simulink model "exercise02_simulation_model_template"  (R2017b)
settings: Solver=ode45  StartTime=0.0  StopTime=10  FixedStep=1e-5  MaxStep=1e-3  RelTol=1e-4  EnableMultiTasking=on
InitFcn:
  | exercise02_simulation_parameters
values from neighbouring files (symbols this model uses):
  cmd_2_newtons_conversion_linear_coefficient = 6.4870e-6    (= 6.487e-06)    [exercise02_get_crazyflie_inner_controller.m]
  cmd_2_newtons_conversion_quadratic_coefficient = 1.3385e-10    [exercise02_get_crazyflie_inner_controller.m]
  cmd_max = 2^16-1    (= 65535)    [exercise02_get_crazyflie_inner_controller.m]
  cmd_min = 0    [exercise02_get_crazyflie_inner_controller.m]
  g = 9.81    [exercise02_get_crazyflie_vehicle_paramters.m]
  K_lqr_outer_loop = K_lqr_outer_loop_discrete_time_200Hz    [exercise02_simulation_parameters.m]
  measurement_noise_accelerometer_covariance_decomposition = U * sqrt(D)    [exercise02_get_measurement_noise_details.m]
  measurement_noise_accelerometer_mean = zeros(3,1)    [exercise02_get_measurement_noise_details.m]
  measurement_noise_accelerometer_seed = randi(measurement_noise_randStream_for_seeds,2^32-1,3,1)    [exercise02_get_measurement_noise_details.m]
  measurement_noise_accelerometer_var = measurement_noise_accelerometer_stddev.^2    [exercise02_get_measurement_noise_details.m]
  measurement_noise_body_accelerations_inclusion_multiplier = 0    [exercise02_get_measurement_noise_details.m]
  measurement_noise_body_rates_inclusion_multiplier = 0    [exercise02_get_measurement_noise_details.m]
  measurement_noise_full_state_covariance_decomposition = U * sqrt(D)    [exercise02_get_measurement_noise_details.m]
  measurement_noise_full_state_inclusion_multiplier = 0    [exercise02_get_measurement_noise_details.m]
  measurement_noise_full_state_mean = [         measurement_noise_p_mean        ;         measurement_noise_p_dot_mean    ;         measurement_noise_psi_mean      ;         measurement_noise_psi_dot_mean        ]    [exercise02_get_measurement_noise_details.m]
  measurement_noise_full_state_seed = [         measurement_noise_p_seed        ;         measurement_noise_p_dot_seed    ;         measurement_noise_psi_seed      ;         measurement_noise_psi_dot_seed        ]    [exercise02_get_measurement_noise_details.m]
  measurement_noise_gyroscope_covariance_decomposition = U * sqrt(D)    [exercise02_get_measurement_noise_details.m]
  measurement_noise_gyroscope_mean = zeros(3,1)    [exercise02_get_measurement_noise_details.m]
  measurement_noise_gyroscope_seed = randi(measurement_noise_randStream_for_seeds,2^32-1,3,1)    [exercise02_get_measurement_noise_details.m]
  measurement_noise_gyroscope_var = measurement_noise_gyroscope_stddev.^2    [exercise02_get_measurement_noise_details.m]
  nrotor_initial_condition = [         nrotor_initial_condition_p          ;         nrotor_initial_condition_p_dot      ;         nrotor_initial_condition_psi        ;         nrotor_initial_condition_psi_dot    ;     ]    [exercise02_get_crazyflie_vehicle_paramters.m]
  nrotor_vehicle_equilibrium_thrust = exercise02_compute_equilibrium_thrusts(nrotor_vehicle_layout_for_controller,nrotor_vehicle_mass_for_controller,g)    [exercise02_simulation_parameters.m]
  nrotor_vehicle_inertia_true = [         16.57 ,   0.83 ,   0.72 ;          0.83 ,  16.66 ,   1.80 ;          0.72 ,   1.80 ,  29.26       ] * 1e-6    [exercise02_get_crazyflie_vehicle_paramters.m]
  nrotor_vehicle_inertia_true_inverse = inv(nrotor_vehicle_inertia_true)    [exercise02_get_crazyflie_vehicle_paramters.m]
  nrotor_vehicle_layout_true = [         [  1 , -1 , -1 ,  1 ] * x_baseline  ;         [ -1 , -1 ,  1 ,  1 ] * y_baseline  ;         [ -1 ,  1 , -1 ,  1 ] * c_baseline        ]    [exercise02_get_crazyflie_vehicle_paramters.m]
  nrotor_vehicle_mass_true = 32e-3    (= 0.032)    [exercise02_get_crazyflie_vehicle_paramters.m]
  nrotor_vehicle_thrust_max = 0.1597*ones( size(nrotor_vehicle_layout_true,2) , 1 )    [exercise02_get_crazyflie_vehicle_paramters.m]
  pid_x_body_rate_integrator_limit = 33.3    [exercise02_get_crazyflie_inner_controller.m]
  pid_x_body_rate_kp = 250.0    (= 250)    [exercise02_get_crazyflie_inner_controller.m]
  pid_y_body_rate_integrator_limit = 33.3    [exercise02_get_crazyflie_inner_controller.m]
  pid_y_body_rate_kp = 250.0    (= 250)    [exercise02_get_crazyflie_inner_controller.m]
  pid_z_body_rate_kp = 120.0    (= 120)    [exercise02_get_crazyflie_inner_controller.m]
  reference_saw_tooth_amplitude_xyz_yaw = [0.3; 0.3; 0.3; 3*deg2rad]    [exercise02_get_reference_specification.m]
  reference_saw_tooth_bias_xyz_yaw = [0.0; 0.0; 0.0; 0*deg2rad]    [exercise02_get_reference_specification.m]
  reference_saw_tooth_inclusion_multiplier = 0    [exercise02_get_reference_specification.m]
  reference_sine_amplitude_xyz_yaw = [0.3; 0.3; 0.3; 3*deg2rad]    [exercise02_get_reference_specification.m]
  reference_sine_bias_xyz_yaw = [0.0; 0.0; 0.0; 0*deg2rad]    [exercise02_get_reference_specification.m]
  reference_sine_period = 5    [exercise02_get_reference_specification.m]
  reference_sine_wave_inclusion_multiplier = 0    [exercise02_get_reference_specification.m]
  reference_step_inclusion_multiplier = 0    [exercise02_get_reference_specification.m]
  reference_step_period = 5    [exercise02_get_reference_specification.m]
  reference_step_xyz_yaw = [0.5; 0.5; 0.5; 10*deg2rad]    [exercise02_get_reference_specification.m]
  sample_time_controller_inner = 1/500    (= 0.002)    [exercise02_simulation_parameters.m]
  sample_time_controller_outer = 1/200    (= 0.005)    [exercise02_simulation_parameters.m]
  sample_time_measurements_body_accelerations = 1/500    (= 0.002)    [exercise02_simulation_parameters.m]
  sample_time_measurements_body_rates = 1/500    (= 0.002)    [exercise02_simulation_parameters.m]
  sample_time_measurements_full_state = 1/200    (= 0.005)    [exercise02_simulation_parameters.m]
undefined symbols (not defined in the file or in its folder): DiscIntNeverNeededParam, sigbuilder_block
libraries: simulink x3
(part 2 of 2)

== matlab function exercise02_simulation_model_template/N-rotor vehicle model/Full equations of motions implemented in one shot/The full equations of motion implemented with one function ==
function [full_state_dot,body_rates,body_accel] = fcn_eom(g,m,J,J_inv,layout,thrusts,full_state)
%
% ----------------------------------------------------------------------- %
% DESCRIPTION:
% This function implements the full equation of motion in one function to
% simplify the exposition.
%
%
% INPUT ARGUMENTS:
% m
% > This is the mass of the vehicle, in units of kilograms
%
% g
% > This is the acceleration due to gravity (typically 9.81), in units of
%   meters per second squared
%
% J
% > This is the moment of inertia matrix of the vehicle (it should be a
%   3-by3 matrix), the units of each element is kilogram meters squared
%
% J_inv
% > This is the inverse of the momement of inertia matrix, it is not
%   compute in this script to reduce the simulation run time slightly
%
% layout
% > This is a matrix that specifies the layout via the following format:
% nrotor_vehicle_layout = [...
%       x_1  ,  x_2  ,  ...  ,  x_{N-1}  ,  x_{N}  ;...
%       y_1  ,  y_2  ,  ...  ,  y_{N-1}  ,  y_{N}  ;...
%       c_1  ,  c_2  ,  ...  ,  c_{N-1}  ,  c_{N}   ...
%   ];
% where:
%   > x_i   is the x coordinate of propeller "i" relative to the CoG
%   > y_i   is the y coordinate of propeller "i" relative to the CoG
%   > c_i   is the thurst to torque coefficient of the propeller, with the
%           sign used to indicate the propeller's direction of rotation,
%           +ve indicates clock-wise propeller rotation.
%
% thrusts
% > This is a colulmn vector with length equal to the number of propellers
%   on the N-rotor vehicle, and each element represents the thrust force in
%   Newtons being produced by the respective propeller
%
% full_state
% > This is a vector of length 12 and is order as:
%   full_state[1:3]     the x,y,z posiiton of the body frame origin
%                       expressed in inertial frame coordinates, in units
%                       of [meters].
%
%   full_state[4:6]     the x,y,z linear velocity of the body frame origin
%                       expressed in inertial frame coordinates, in units
%                       of [meters per second].
%
%   full_state[7:9]     the roll, pitch, and yaw intrinsic Euler angles
%                       respectively, in units of [radians].
%
%   full_state[10:12]   the angular velocity of the roll, pitch, and yaw
%                       intrinsic Euler angles respectively, in units of
%                       [radians per second].
%
%
% RETURN ARGUMENTS:
% full_state_dot
% > This is a vector of length 12 and is ordered as:
%   full_state_dot[1:3]
%      - This is position dot and is taken directly as full_state[4:6]
%
%   full_state_dot[4:6]
%      - This is the position double dot and is computed using the equation
%        of motion for transaltion, it has units of [meters per second
%        squared]
%
%   full_state_dot[7:9]
%      - This is the angular velocity of the intrinsic Euler angles and is
%        taken directly as full_state[10:12]
%
%   full_state_dot[10:12]
%      - This is the angular accelerations of the intrinsic Euler angles
%        and is computed using the equation of motion for Euler angle
%        rotations, it has units of [radians per second squared]
%
% body_rates
% > This is a vector of length 3, each element represents the angular
%   velocity of the body frame as measured about the body frame's
%   coordinate axes, ordered as:
%   body_rates = [ w_x ; w_y ; w_z ];
%   In other words, this is exactly what is measured by a typical
%   strap-down Inertial Measurement Unit (IMU) that is attached to the body
%   of most all flying vehicles. It is computed directly from the "psi_dot"
%   by that is extracted from the "full_state" by applying the
%   transformation matrix "T". It has units of [radians per second];
%
% body_accel
% > This is a vector of length 3, each element represents the linear
%   accelerations of the body frame as measured along the body frame's
%   coordinate axes, i.e., this is exctly what is measured by a typical
%   strap-down Inertial Measurement Unit (IMU). It is computed directly
%   from the "pos_double_dot" by applying the rotation matrix from inertial
%   to body frame. It has units of [meters per second squared].
%
% ----------------------------------------------------------------------- %


% Extract the components of the full state
%pos      =  full_state(1:3);
pos_dot  =  full_state(4:6);
psi      =  full_state(7:9);
psi_dot  =  full_state(10:12);


% Extract each Euler angles
roll   =  psi(1);  % Roll  (gamma is the symbol used in the script)
pitch  =  psi(2);  % Pitch (beta  is the symbol used in the script)
yaw    =  psi(3);  % Yaw   (alpha is the symbol used in the script)


% Extract each Euler anglular rates
roll_dot   =  psi_dot(1);  % Roll  angular velocity
pitch_dot  =  psi_dot(2);  % Pitch angular velocity
%yaw_dot    =  psi_dot(3); % Yaw   angular velocity, not needed


% Compute the rotation matrix from body frame to inertial frame:
R_B2I = [...
            cos(yaw)*cos(pitch)  ,...
                cos(yaw)*sin(pitch)*sin(roll)-sin(yaw)*cos(roll)  ,...
                cos(yaw)*sin(pitch)*cos(roll)+sin(yaw)*sin(roll)   ...
            ;...
            sin(yaw)*cos(pitch)  ,...
                sin(yaw)*sin(pitch)*sin(roll)+cos(yaw)*cos(roll)  ,...
                sin(yaw)*sin(pitch)*cos(roll)-cos(yaw)*sin(roll)   ...
            ;...
            -sin(pitch)  ,...
                cos(pitch)*sin(roll)  ,...
                cos(pitch)*cos(roll)   ...
    ];


% Compute the T matrix:
T = [...
        1  ,  0          ,  -sin(pitch)            ;...
        0  ,  cos(roll)  ,   sin(roll)*cos(pitch)  ;...
        0  , -sin(roll)  ,   cos(roll)*cos(pitch)   ...
    ];


% Compute the T inverse matrix:
T_inv = [...
        1  ,  sin(roll)*tan(pitch)  ,   cos(roll)*tan(pitch)  ;...
        0  ,  cos(roll)             ,  -sin(roll)             ;...
        0  ,  sin(roll)*sec(pitch)  ,   cos(roll)*sec(pitch)   ...
    ];


% Compute the time derivative of the T matrix:
T_dot = [...
        0  ,   0                   ,  -pitch_dot*cos(pitch)                                          ;...
        0  ,  -roll_dot*sin(roll)  ,   roll_dot*cos(roll)*cos(pitch)-pitch_dot*sin(roll)*sin(pitch)  ;...
        0  ,  -roll_dot*cos(roll)  ,  -roll_dot*sin(roll)*cos(pitch)-pitch_dot*cos(roll)*sin(pitch)   ...
    ];


% Implement the equation of motion for translation
pos_double_dot = (1/m) .* ( R_B2I * [0;0;sum(thrusts(:))] ) + [0;0;-g];


% Compute the body rates from the Euler angluar rates
w = T * psi_dot;


% Implement the equation of motion for body frame rotations
w_dot = J_inv * ( [layout(2,:);-layout(1,:);layout(3,:)] * thrusts - cross( w , J*w ) );


% Implement the equation of motion for Euler angle rotations
psi_double_dot = T_inv * ( w_dot - T_dot * psi_dot );


% Put together the "full_state_dot" return variable
full_state_dot = [...
        pos_dot ;...
        pos_double_dot ;...
        psi_dot ;...
        psi_double_dot ...
    ];


% Put together the "body_rates" return variable
body_rates = w;


% Finally compute the accelerations in the body frame
% > by "simply" rotating the inertial frame linear accelerations, i.e.,
%   "pos_double_dot", from the inertial frame into the body frame
% > do you need to account for the fact that the body frame accelerations
%   are measured in a rotating frame?
body_accel = transpose(R_B2I) * psi_double_dot;


end

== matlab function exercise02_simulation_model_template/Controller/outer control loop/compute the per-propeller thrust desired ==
function thrusts_per_motor = compute_per_motor_thrust( thrusts_for_equilibrium , additional_thrust_desired )
% ----------------------------------------------------------------------- %
% DESCRIPTION:
% This function computes the desired thrust per propeller that provides the
% total thrust and body frame (x,y,z) torques requested for an N-rotor
% vehicle with a particular layout
%
%
% INPUT ARGUMENTS:
% thrusts_for_equilibrium
% > This is a colulmn vector with length equal to the number of propellers
%   on the N-rotor vehicle, and each element represents the thrust force in
%   Newtons that will maintain the N-rotor vehicle at the hover equilibrium
%
% additional_thrust_desired [Newtons]
% > This is the total additional thrust force desired
%
%
% RETURN ARGUMENTS:
% thrusts_per_motor
% > This is a colulmn vector with length equal to the number of propellers
%   on the N-rotor vehicle, and each element represents the thrust force in
%   Newtons that is desired from the respective propeller
%
%
% ----------------------------------------------------------------------- %

% Compute any residual thrust that results from the "thrusts_for_torque"
total_equilibrium_thrust = sum( thrusts_for_equilibrium(:) );

% Compute the desired thrust per propeller:
thrusts_per_motor = thrusts_for_equilibrium * ...
    ( (additional_thrust_desired+total_equilibrium_thrust)/total_equilibrium_thrust );

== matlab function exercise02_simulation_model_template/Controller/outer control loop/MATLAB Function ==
function xy_error_in_body_frame = rotate_xy_intertial_to_body( current_yaw , xy_error_in_inertial_frame )
% ----------------------------------------------------------------------- %
% DESCRIPTION:
% This function rotates an (x,y) coordainte and (x_dot,y_dot) velocity
% vector from the interial frame into (approximately) the body frame. The
% approximate is because the rotation into the body frame is only based on
% the current yaw of the vehicle and assumes that roll and pitch are zero.
%
%
% INPUT ARGUMENTS:
% current_yaw
% > The intrinsic Euler yaw angle, in radians
%
% xy_error_in_inertial_frame [m;m;m/s;m/s]
% > The measurement of (x,y) position and velocities in the inertial frame
%
%
% RETURN ARGUMENTS:
% xy_error_in_body_frame
% > The measurement of (x,y) position and velocities rotated into the body
%   frame
%
%
% ----------------------------------------------------------------------- %


% Extract the inertial position and velocities
x_I      =  xy_error_in_inertial_frame(1);
y_I      =  xy_error_in_inertial_frame(2);
xdot_I   =  xy_error_in_inertial_frame(3);
ydot_I   =  xy_error_in_inertial_frame(4);


% Initialise the return variable "xy_error_in_body_frame" to zeros
% > This can be required so that Simulink knows the expected size
xy_error_in_body_frame = zeros(4,1);


% Rotate the inertial POSITIONS into the body frame
% > For computing x in the body frame
xy_error_in_body_frame(1,1) =  +x_I;
% > For computing y in the body frame
xy_error_in_body_frame(2,1) =  +y_I;


% Rotate the inertial VELOCITIES into the body frame
% > For computing xdot in the body frame
xy_error_in_body_frame(3,1) =  +xdot_I;
% > For computing ydot in the body frame
xy_error_in_body_frame(4,1) =  +ydot_I;
